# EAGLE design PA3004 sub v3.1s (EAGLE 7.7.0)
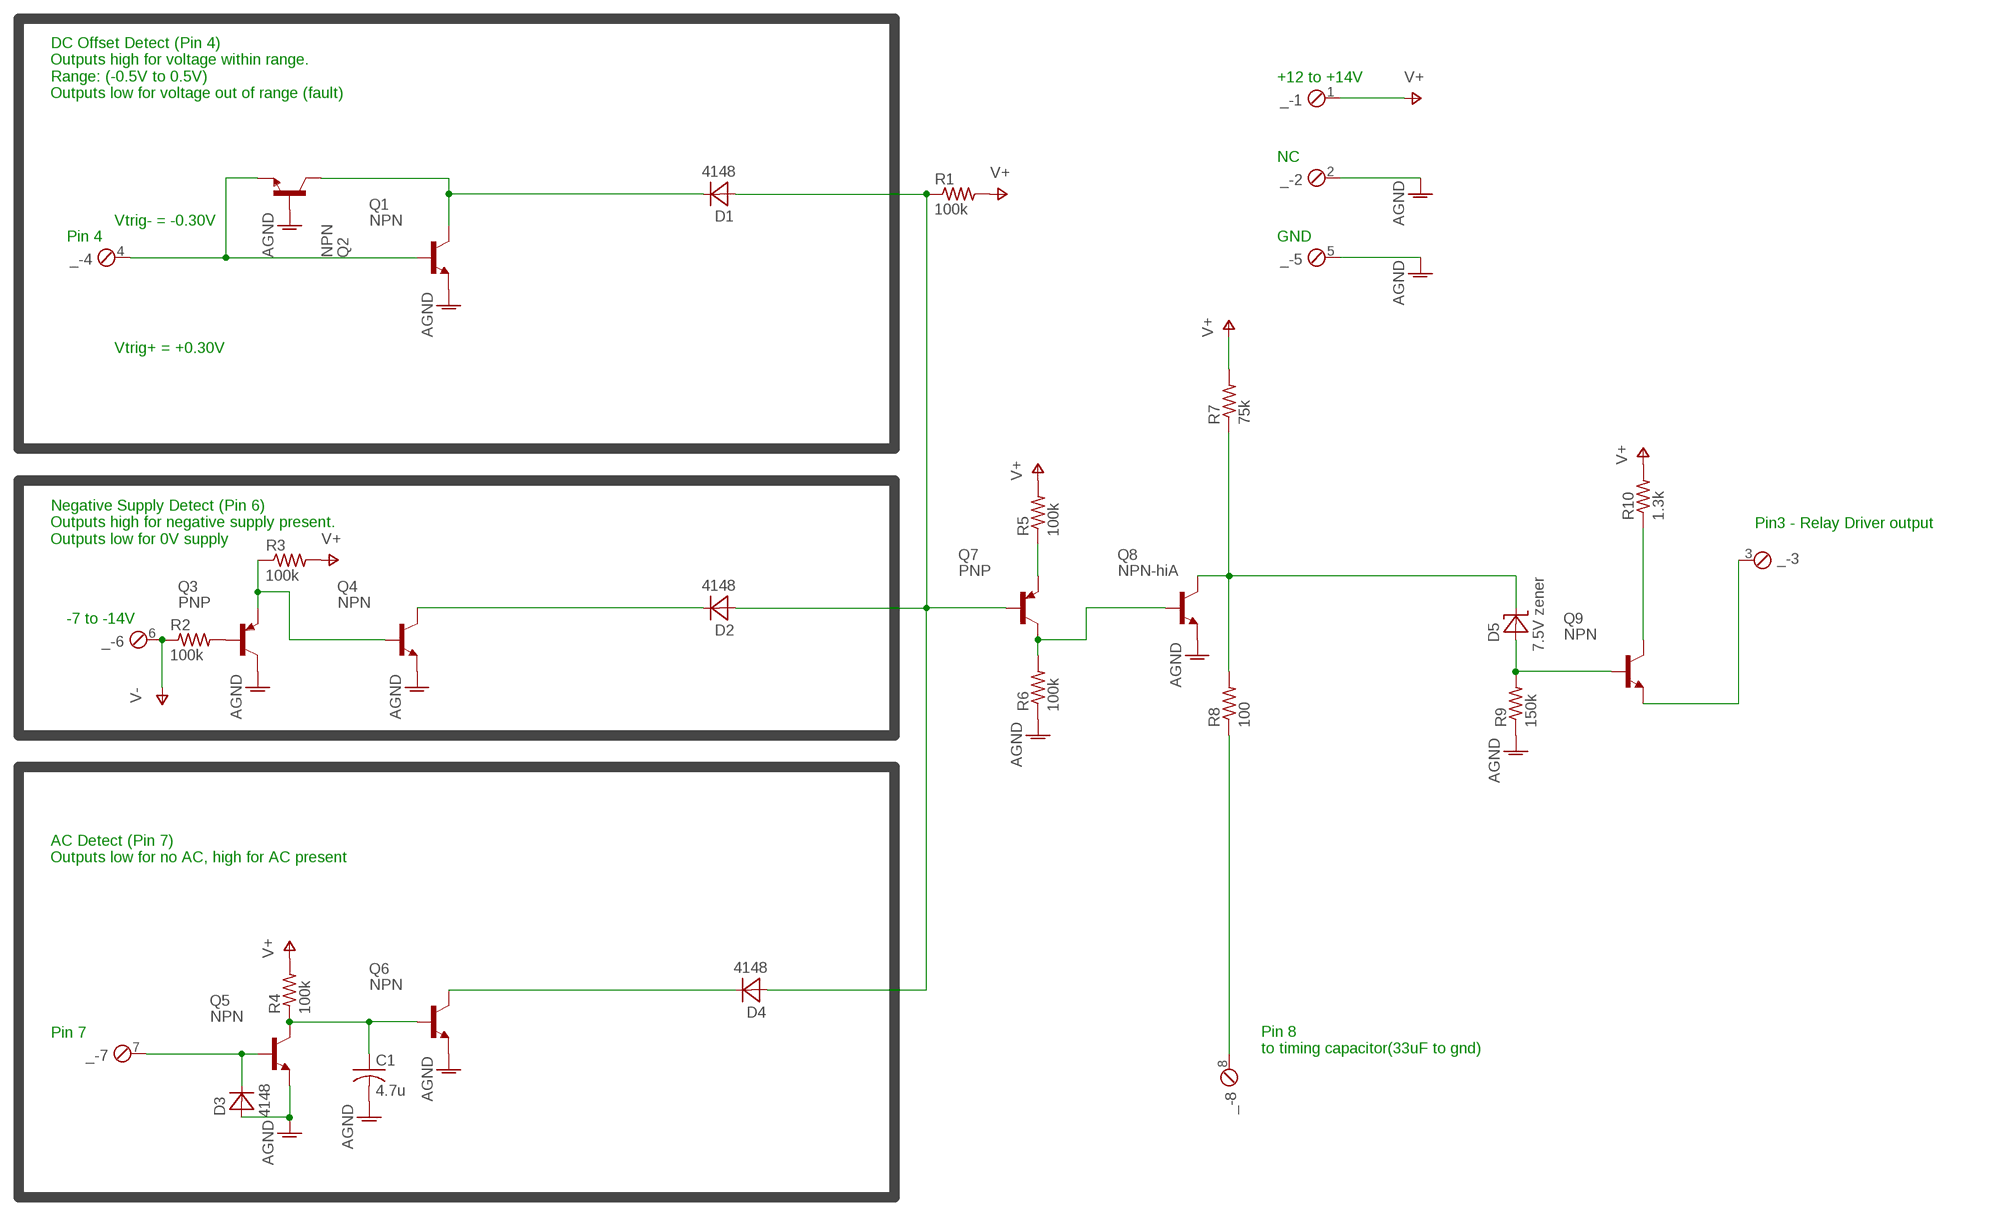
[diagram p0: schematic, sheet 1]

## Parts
_  MPT8  [8POL254]
C1  4.7u  C-USC0603  [C0603]
D1  4148  4148_SMD0603  [D0603]
D2  4148  4148_SMD0603  [D0603]
D3  4148  4148_SMD0603  [D0603]
D4  4148  4148_SMD0603  [D0603]
D5  7.5V zener  DIODE_Z_CZRF52C5V1  [D0805]
Q1  NPN  FJV1845FMTF  [SOT-23-3]
Q2  NPN  FJV1845FMTF  [SOT-23-3]
Q3  PNP  FJV992FMTF  [SOT-23-3]
Q4  NPN  FJV1845FMTF  [SOT-23-3]
Q5  NPN  FJV1845FMTF  [SOT-23-3]
Q6  NPN  FJV1845FMTF  [SOT-23-3]
Q7  PNP  FJV992FMTF  [SOT-23-3]
Q8  NPN-hiA  FJV1845FMTF  [SOT-23-3]
Q9  NPN  FJV1845FMTF  [SOT-23-3]
R1  100k  R-US_R0603  [R0603]
R2  100k  R-US_R0603  [R0603]
R3  100k  R-US_R0603  [R0603]
R4  100k  R-US_R0603  [R0603]
R5  100k  R-US_R0603  [R0603]
R6  100k  R-US_R0603  [R0603]
R7  75k  R-US_R0603  [R0603]
R8  100  R-US_R0603  [R0603]
R9  150k  R-US_R0603  [R0603]
R10  1.3k  R-US_R0603  [R0603]

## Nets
-12V: _.6 R2.1 ; supply symbol labelled V-
AGND: _.2 _.5 C1.2 D3.A Q1.2(E) Q2.1(B) Q3.3(C) Q4.2(E) Q5.2(E) Q6.2(E) Q8.2(E) R6.1 R9.1
N$1: _.4 Q1.1(B) Q2.2(E)
N$2: D1.C Q1.3(C) Q2.3(C)
N$3: D1.A D2.A D4.A Q7.1(B) R1.1
N$4: D4.C Q6.3(C)
N$5: Q3.1(B) R2.2
N$6: Q7.3(C) Q8.1(B) R6.2
N$7: _.7 D3.C Q5.1(B)
N$8: Q7.2(E) R5.1
N$9: C1.1 Q5.3(C) Q6.1(B) R4.1
N$10: Q3.2(E) Q4.1(B) R3.1
N$11: _.8 R8.1
N$12: D5.2(A) Q9.1(B) R9.2
N$13: D5.1(C) Q8.3(C) R7.1 R8.2
N$14: Q9.3(C) R10.1
N$15: D2.C Q4.3(C)
N$16: _.3 Q9.2(E)
V+: _.1 R1.2 R3.2 R4.2 R5.2 R7.2 R10.2

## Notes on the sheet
- +12 to +14V
- DC Offset Detect (Pin 4)
  Outputs high for voltage within range.
  Range: (-0.5V to 0.5V) 
  Outputs low for voltage out of range (fault)
- NC
- Vtrig- = -0.30V
- Pin 4 | GND
- Vtrig+ = +0.30V
- Pin3 - Relay Driver output
- Negative Supply Detect (Pin 6)
  Outputs high for negative supply present. 
  Outputs low for 0V supply
- -7 to -14V
- AC Detect (Pin 7)
  Outputs low for no AC, high for AC present
- Pin 7
- Pin 8
  to timing capacitor(33uF to gnd)

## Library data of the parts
_ = con-phoenix-254:MPT8: PHOENIX CONNECTOR; OC_FARNELL: unknown; OC_NEWARK: unknown
C1 = rcl:C-US: CAPACITOR, American symbol
D1-D4 = PA3004 Components:4148_SMD0603: 4148 Diode, 0603 footprint
D5 = PA3004 Components:DIODE_Z_CZRF52C5V1: Zener Diode - SMD footprint 0805
Q1 Q2 Q4-Q6 Q8 Q9 = PA3004 Components:FJV1845FMTF: NPN Transistor - SMD SOT 23 Mouser#: 512-FJV1845FMTF
Q3 Q7 = PA3004 Components:FJV992FMTF: PNP Transistor - SMD SOT 23-3
R1-R10 = rcl:R-US_: RESISTOR, American symbol

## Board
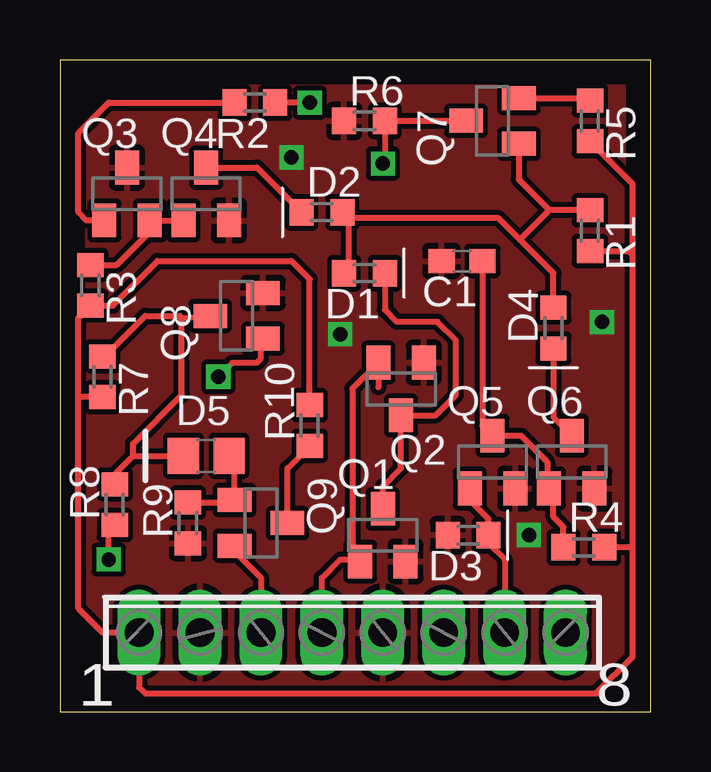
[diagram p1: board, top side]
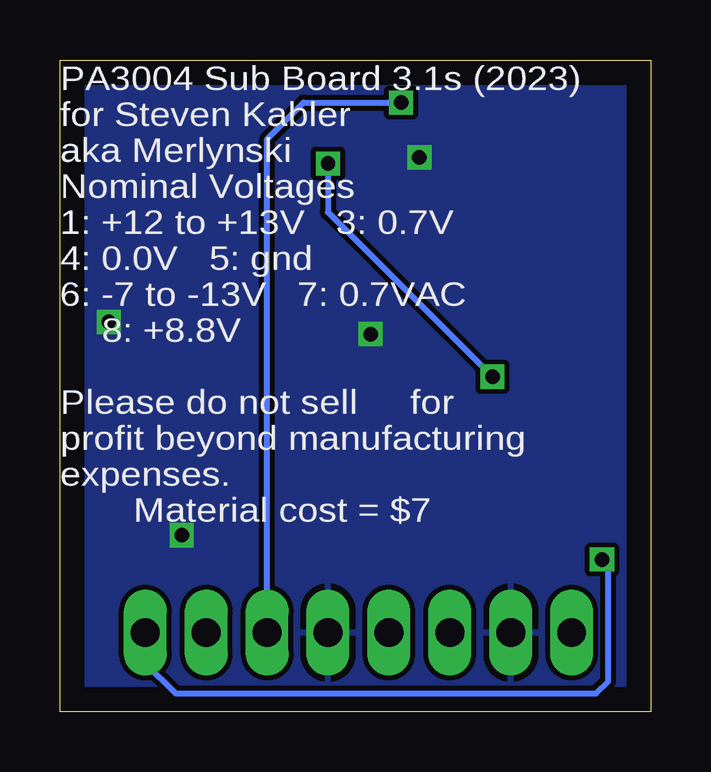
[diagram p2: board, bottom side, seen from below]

Size 24.64 x 27.18 mm. Coordinates in mm from the lower left corner, seen from the top.
Outline: 0,0 24.64,0 24.64,27.18 0,27.18 0,0
Copper layers (1*16): Top 0.035mm / dielectric 1.5mm / Bottom 0.035mm
Design rules "default": minimum track width 10mil, minimum drill 24mil, track to track 8mil, track to pad 8mil, pad to pad 8mil, via to via 8mil, smd to smd 8mil, copper to edge 40mil, drill to drill 8mil, minimum pad ring 10mil, minimum via ring 8mil, stop-mask expansion 4mil, vias tented up to drill 0mil, thermal gap 10mil

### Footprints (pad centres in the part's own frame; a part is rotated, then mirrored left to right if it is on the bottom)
8POL254 = drill 1.2 long: 1 -8.89,0; 2 -6.35,0; 3 -3.81,0; 4 -1.27,0; 5 1.27,0; 6 3.81,0; 7 6.35,0; 8 8.89,0
C0603 = smd 1.1 x 1: 1 -0.85,0; 2 0.85,0
D0603 = smd 1 x 1.1: A 0.85,0; C -0.85,0
D0805 = smd 1.3 x 1.5: 1 -0.95,0; 2 0.95,0
SOT-23-3 = smd 1 x 1.4: 1 -0.95,-1.1; 2 0.95,-1.1; 3 0,1.1
R0603 = smd 1 x 1.1: 1 -0.85,0; 2 0.85,0

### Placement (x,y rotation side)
_  12.19,3.3 0 top
C1  16.76,18.8 180 top
D1  12.7,18.29 180 top
D2  10.92,20.83 0 top
D3  17.02,7.37 180 top
D4  20.57,16 90 top
D5  6.1,10.67 0 top
Q1  13.46,7.37 0 top
Q2  14.22,13.46 180 top
Q3  2.79,21.59 0 top
Q4  6.1,21.59 0 top
Q5  18.03,10.41 0 top
Q6  21.34,10.41 0 top
Q7  18.03,24.64 90 top
Q8  7.37,16.51 90 top
Q9  8.38,7.87 270 top
R1  22.1,20.07 270 top
R2  8.13,25.4 180 top
R3  1.27,17.78 270 top
R4  21.84,6.86 0 top
R5  22.1,24.64 270 top
R6  12.7,24.64 0 top
R7  1.78,13.97 270 top
R8  2.29,8.64 90 top
R9  5.33,7.87 90 top
R10  10.41,11.94 90 top

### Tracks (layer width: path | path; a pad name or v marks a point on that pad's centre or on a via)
-12V  (via drill 0.6)
  Top 0.254: v10.41,25.4 R2.1
  Bottom 0.254: _.6 16,23.88 14.48,25.4 v10.41,25.4
AGND  (via drill 0.6)
  other vias: 19.56,7.37 11.68,15.75 9.65,23.11 22.61,16.26
  pour Top: 0,0 0,27.18 24.64,27.18 24.64,0
  pour Bottom: 0,0 24.64,0 24.64,27.18 0,27.18
N$1
  Top 0.254: _.4 10.92,5.59 11.68,6.35 12.43,6.35 Q1.1 12.19,6.59 12.19,13.48 Q2.2 13.27,13.53
N$2
  Top 0.254: Q1.3 13.46,9.4 14.22,10.16 Q2.3 15.66,12.36 16.51,13.21 16.51,15.49 15.75,16.26 14.06,16.26 13.55,16.76 D1.C
N$3
  Top 0.254: D4.A 20.57,18.29 19.18,19.68 | 19.18,19.68 18.29,20.57 12.03,20.57 | R1.1 20.41,20.92 | 20.41,20.92 19.18,19.68 | Q7.1 19.13,22.19 20.41,20.92 | 12.03,20.57 D2.A | 12.03,20.57 12.03,18.46 D1.A
N$4
  Top 0.254: D4.C 20.57,12.28 Q6.3
N$5
  Top 0.254: Q3.1 1.1,20.49 0.76,20.83 0.76,24.13 2.03,25.4 R2.2
N$6  (via drill 0.6)
  Top 0.254: v6.6,13.97 7.2,14.56 8.21,14.56 8.38,14.73 8.38,15.48 Q8.1 | Q7.3 R6.2 13.55,22.95 v13.46,22.86
  Bottom 0.254: v13.46,22.86 13.46,20.83 v6.6,13.97
N$7
  Top 0.254: _.7 18.54,6.35 17.87,7.02 D3.C 17.87,8.04 17.27,8.64 17.27,9.13 Q5.1
N$8
  Top 0.254: Q7.2 22,25.59 R5.1
N$9
  Top 0.254: R4.1 20.99,7.71 20.57,8.13 20.57,9.13 Q6.1 20.32,9.38 20.32,10.41 19.22,11.51 Q5.3 17.61,11.93 C1.1
N$10
  Top 0.254: Q4.1 Q3.2 3.56,20.3 3.56,19.81 2.37,18.63 R3.1
N$11  (via drill 0.6)
  Top 0.254: v2.03,6.35 2.03,7.53 R8.1
  Bottom 0.254: _.8 21.08,2.03 19.81,0.76 2.29,0.76 1.78,1.27 1.78,6.1 v2.03,6.35
N$12
  Top 0.254: R9.2 7.18,8.72 Q9.1 7.28,10.43 D5.2
N$13
  Top 0.254: R8.2 2.29,9.91 3.05,10.67 | 3.05,10.67 D5.1 | R7.1 1.87,14.82 3.56,16.51 5,16.51 5.08,16.43 | 3.05,10.67 3.05,11.18 5.08,13.21 5.08,16.43 | 5.08,16.43 Q8.3
N$14
  Top 0.254: Q9.3 9.48,10.16 R10.1
N$15
  Top 0.254: Q4.3 8.21,22.69 D2.C
N$16
  Top 0.254: Q9.2 7.28,6.69 8.38,5.59 _.3
V+
  Top 0.254: 23.88,6.86 23.88,2.29 22.35,0.76 3.56,0.76 3.3,1.02 _.1 1.78,3.3 0.76,4.32 0.76,13.21 | 23.88,6.86 R4.2 | R10.2 10.41,18.03 9.65,18.8 4.06,18.8 2.2,16.93 R3.2 0.76,16.42 0.76,13.21 | 23.88,6.86 23.88,19.05 | 23.88,19.05 23.88,22.01 R5.2 | R1.2 23.71,19.22 23.88,19.05 | R7.2 0.85,13.12 0.76,13.21

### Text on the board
tNames: 1 | 8
bNames: PA3004 Sub Board 3.1s (2023) / for Steven Kabler / aka Merlynski / Nominal Voltages / 1: +12 to +13V 3: 0.7V / 4: 0.0V 5: gnd / 6: -7 to -13V 7: 0.7VAC / 8: +8.8V / / Please do not sell for / profit beyond manufacturing / expenses. / Material cost = $7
